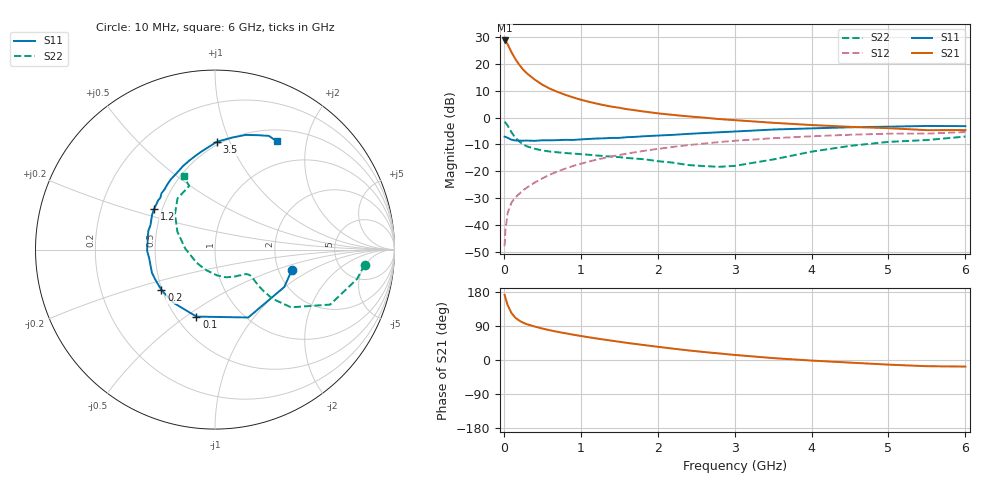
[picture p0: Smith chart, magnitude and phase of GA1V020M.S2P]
! Infineon Technologies  Discrete & RF Semiconductors
! BF775
! Si NPN RF Bipolar Junction Transistor in SOT23
! VCE = 1 V  IC = 20 mA
! Common Emitter S-Parameters:  May  1996
# GHz  S  MA  R  50
!  f  S11  S21  S12  S22
! GHz  MAG  ANG  MAG  ANG  MAG  ANG  MAG  ANG
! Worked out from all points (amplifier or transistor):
!   36 points, 10 MHz to 6 GHz, reference 50 ohm
!   highest |S21| = 28.8 dB at 10 MHz (marker M1)
!   |S21| within 3 dB of that: start of sweep to 76.03 MHz
!   unconditionally stable (mu >= 1): start of sweep to 11.52 MHz; 175.5 MHz to end of sweep
!   at 250 MHz: K = 1.17, MAG = 20.0 dB, |S12| = -27.1 dB
!   at 1.4 GHz: K = 1.39, MAG = 5.6 dB, |S12| = -14.5 dB
!   at 6 GHz: K = 1.11, MAG = -1.7 dB, |S12| = -5.4 dB
!   S11 on the Smith chart (normalised r, x): 10 MHz: 2.37, -0.66; 100 MHz: 0.63, -0.55; 200 MHz: 0.50, -0.26; 1.2 GHz: 0.45, +0.24; 3.5 GHz: 0.48, +0.90; 6 GHz: 0.65, +1.53
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0.01  0.4435 -14.6  27.62 171.9  0.004 84.3  0.8378 -5.8
0.02  0.4387 -28.3  26.95 164.1  0.0078 76.0  0.808 -11.7
0.05  0.4212 -63.9  23.3 144.6  0.0167 68.6  0.7111 -25.5
0.1  0.3873 -105.5  16.64 123.6  0.0261 60.1  0.532 -37.2
0.15  0.376 -128.3  12.43 111.5  0.0325 58.5  0.4219 -40.5
0.2  0.3739 -143.0  9.762 104.0  0.0379 60.0  0.3597 -40.5
0.25  0.3722 -153.3  7.907 98.5  0.044 61.4  0.3164 -39.8
0.3  0.3743 -159.9  6.711 94.4  0.0496 63.7  0.292 -38.7
0.4  0.3697 -172.2  5.159 88.4  0.0614 65.7  0.2635 -37.1
0.5  0.3785 -179.2  4.125 83.0  0.0736 66.5  0.2448 -36.3
0.6  0.3775 174.6  3.469 78.4  0.0867 66.8  0.2331 -36.6
0.7  0.3813 169.0  3.022 74.2  0.0993 66.9  0.2256 -37.4
0.9  0.3844 159.3  2.392 66.9  0.1256 65.5  0.2137 -40.1
1.1  0.4004 151.1  1.989 60.2  0.1511 63.9  0.2034 -44.7
1.2  0.4081 146.4  1.841 56.9  0.1639 62.9  0.1972 -47.0
1.6  0.4327 133.6  1.443 45.2  0.2135 57.9  0.1772 -59.1
2.2  0.4781 116.1  1.127 30.0  0.2849 49.6  0.1447 -85.0
2.8  0.5343 101.6  0.942 17.3  0.3504 40.6  0.1212 -129.1
3.5  0.601 89.0  0.803 5.0  0.4134 29.7  0.166 178.0
4.5  0.6617 75.0  0.675 -6.9  0.4806 15.1  0.2979 138.5
5.5  0.7009 64.7  0.585 -16.4  0.5047 1.2  0.3825 112.1
6  0.695 60.1  0.587 -17.3  0.5387 -2.8  0.4441 113.1
